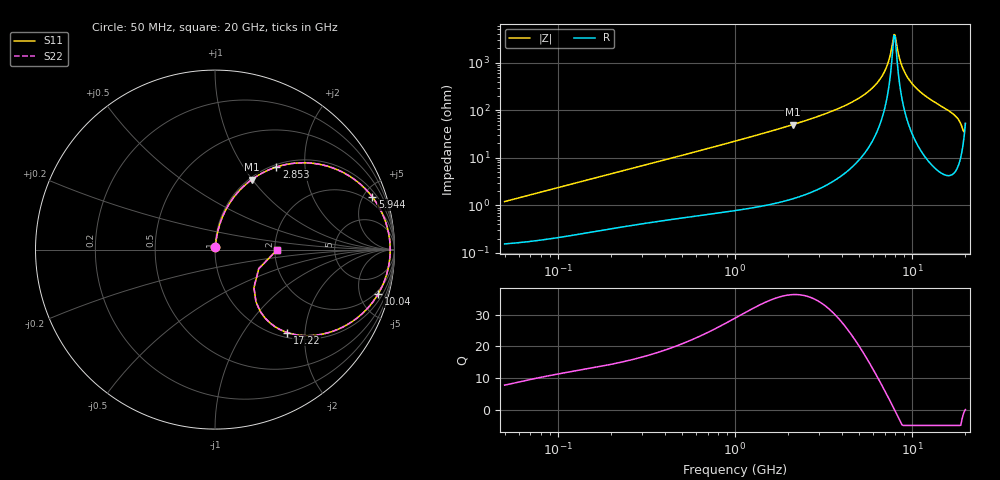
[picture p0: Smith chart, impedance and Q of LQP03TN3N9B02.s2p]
!Murata Part Number: LQP03TN3N9B02
!These Parameters are Measured in Series Mode Connection
!  o--[Z]--o
!Port1  Port2
!  o-------o
!Freq. Start=50[MHz] Stop=20[GHz], 401[Steps]
# Hz S RI R 50
!Freq.(Hz) S11(Real) S11(Imag) S21(Real) S21(Imag) S12(Real) S12(Imag) S22(Real) S22(Imag)
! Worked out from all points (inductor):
!   401 points, 50 MHz to 20 GHz, reference 50 ohm
!   read as one part in series: L = 3.78 nH near 51.52 MHz
!   highest Q = 36.3 at 2.115 GHz (marker M1), where L = 3.74 nH
!   self-resonance near 7.902 GHz
!   S11 on the Smith chart (normalised r, x): 50 MHz: 1.00, +0.02; 2.853 GHz: 1.04, +1.43; 5.944 GHz: 1.44, +5.79; 10.04 GHz: 1.62, -7.10; 17.22 GHz: 1.09, -1.62; 20 GHz: 2.06, -0.01
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5e7  0.00168 0.0119  0.9983 -0.0119  0.9983 -0.0119  0.00168 0.0119
1.364002e8  0.00352 0.0316  0.9965 -0.0316  0.9965 -0.0316  0.00352 0.0316
3.721004e8  0.0115 0.0825  0.9885 -0.0825  0.9885 -0.0825  0.0115 0.0825
1e9  0.0542 0.2097  0.9458 -0.2097  0.9458 -0.2097  0.0542 0.2097
2.114743e9  0.2043 0.3896  0.7957 -0.3896  0.7957 -0.3896  0.2043 0.3896
2.728004e9  0.3168 0.4513  0.6832 -0.4513  0.6832 -0.4513  0.3168 0.4513
2.853386e9  0.3414 0.46  0.6586 -0.46  0.6586 -0.46  0.3414 0.46
4.275624e9  0.6253 0.4649  0.3747 -0.4649  0.3747 -0.4649  0.6253 0.4649
5.944466e9  0.8766 0.2934  0.1234 -0.2934  0.1234 -0.2934  0.8766 0.2934
6.802353e9  0.9455 0.1688  0.0545 -0.1688  0.0545 -0.1688  0.9455 0.1688
7.442007e9  0.9705 0.0735  0.0295 -0.0735  0.0295 -0.0735  0.9705 0.0735
7.784049e9  0.9756 0.0239  0.0244 -0.0239  0.0244 -0.0239  0.9756 0.0239
8.020766e9  0.9762 -0.00959  0.0238 0.00959  0.0238 0.00959  0.9762 -0.00959
8.141811e9  0.9756 -0.0263  0.0244 0.0263  0.0244 0.0263  0.9756 -0.0263
8.516016e9  0.9704 -0.0764  0.0296 0.0764  0.0296 0.0764  0.9704 -0.0764
8.907419e9  0.96 -0.1256  0.04 0.1256  0.04 0.1256  0.96 -0.1256
1.004137e10  0.9086 -0.2479  0.0914 0.2479  0.0914 0.2479  0.9086 -0.2479
1.334722e10  0.6841 -0.4445  0.3159 0.4445  0.3159 0.4445  0.6841 -0.4445
1.721783e10  0.4023 -0.4621  0.5977 0.4621  0.5977 0.4621  0.4023 -0.4621
1.855685e10  0.28 -0.3828  0.72 0.3828  0.72 0.3828  0.28 -0.3828
1.912117e10  0.2279 -0.2902  0.7721 0.2902  0.7721 0.2902  0.2279 -0.2902
2e10  0.3456 -0.0022  0.6544 0.0022  0.6544 0.0022  0.3456 -0.0022
